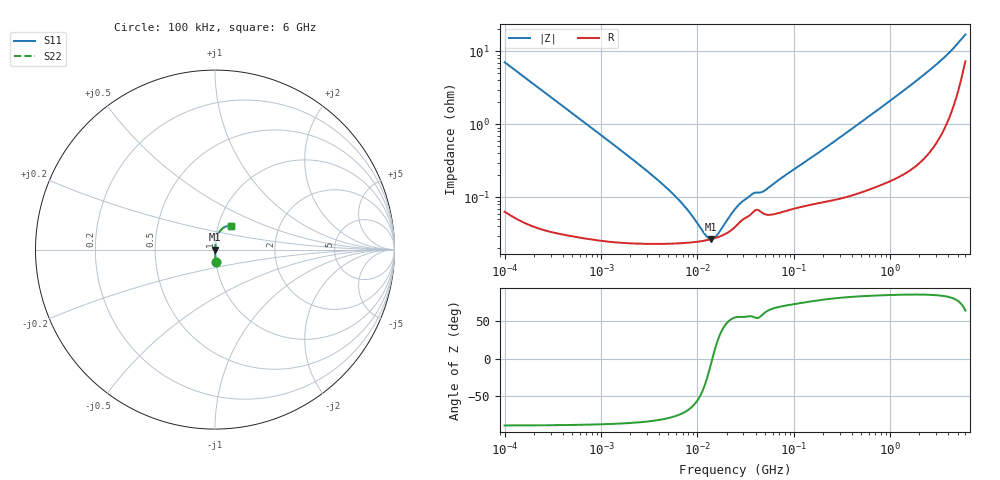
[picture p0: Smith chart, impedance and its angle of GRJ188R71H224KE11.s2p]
!Murata Part Number: GRJ188R71H224KE11
!These Parameters are Measured in Series Mode Connection
!Data Generated on Jun 19, 2026
!  o--ll--o
!Port1  Port2
!  o------o
!Operation Temp=25[degC], DC Bias Voltage=0[V]
!Freq. Start=100[kHz] Stop=6[GHz] 401[Steps]
# Hz S RI R 50
!Freq.(Hz) S11(Real) S11(Imag) S21(Real) S21(Imag) S12(Real) S12(Imag) S22(Real) S22(Imag)
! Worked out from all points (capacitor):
!   401 points, 100 kHz to 6 GHz, reference 50 ohm
!   read as one part in series: C = 224 nF near 105.7 kHz
!   lowest |Z| = 26.9 mohm at 13.75 MHz (marker M1)
!   series resonance near 14.25 MHz, so ESL is about 560 pH
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100000  0.00565 -0.0706  0.9944 0.0706  0.9944 0.0706  0.00565 -0.0706
222032  0.0014 -0.032  0.9986 0.032  0.9986 0.032  0.0014 -0.032
631452  0.000405 -0.0113  0.9996 0.0113  0.9996 0.0113  0.000405 -0.0113
2060590  0.000246 -0.0034  0.9998 0.0034  0.9998 0.0034  0.000246 -0.0034
3987316  0.000233 -0.00166  0.9998 0.00166  0.9998 0.00166  0.000233 -0.00166
6911753  0.000236 -0.000793  0.9998 0.000793  0.9998 0.000793  0.000236 -0.000793
8612937  0.000241 -0.000528  0.9998 0.000528  0.9998 0.000528  0.000241 -0.000528
1.198108e7  0.000256 -0.000175  0.9997 0.000175  0.9997 0.000175  0.000256 -0.000175
1.301164e7  0.000262 -9.16e-05  0.9997 9.16e-05  0.9997 9.16e-05  0.000262 -9.16e-05
1.374747e7  0.000267 -3.62e-05  0.9997 3.62e-05  0.9997 3.62e-05  0.000267 -3.62e-05
1.492997e7  0.000275 4.7e-05  0.9997 -4.7e-05  0.9997 -4.7e-05  0.000275 4.7e-05
1.621418e7  0.000284 0.000131  0.9997 -0.000131  0.9997 -0.000131  0.000284 0.000131
2.517799e7  0.000407 0.000596  0.9996 -0.000596  0.9996 -0.000596  0.000407 0.000596
2.889002e7  0.000487 0.000718  0.9995 -0.000718  0.9995 -0.000718  0.000487 0.000718
3.700465e7  0.000611 0.000924  0.9994 -0.000924  0.9994 -0.000924  0.000611 0.000924
5.007898e7  0.000588 0.0011  0.9994 -0.0011  0.9994 -0.0011  0.000588 0.0011
1.546735e8  0.000809 0.00347  0.9992 -0.00347  0.9992 -0.00347  0.000809 0.00347
9.76689e8  0.00207 0.0206  0.9979 -0.0206  0.9979 -0.0206  0.00207 0.0206
2.229039e9  0.00561 0.0473  0.9944 -0.0473  0.9944 -0.0473  0.00561 0.0473
3.759065e9  0.0166 0.0838  0.9834 -0.0838  0.9834 -0.0838  0.0166 0.0838
4.814911e9  0.0356 0.1123  0.9644 -0.1123  0.9644 -0.1123  0.0356 0.1123
6e9  0.0869 0.1311  0.9131 -0.1311  0.9131 -0.1311  0.0869 0.1311
